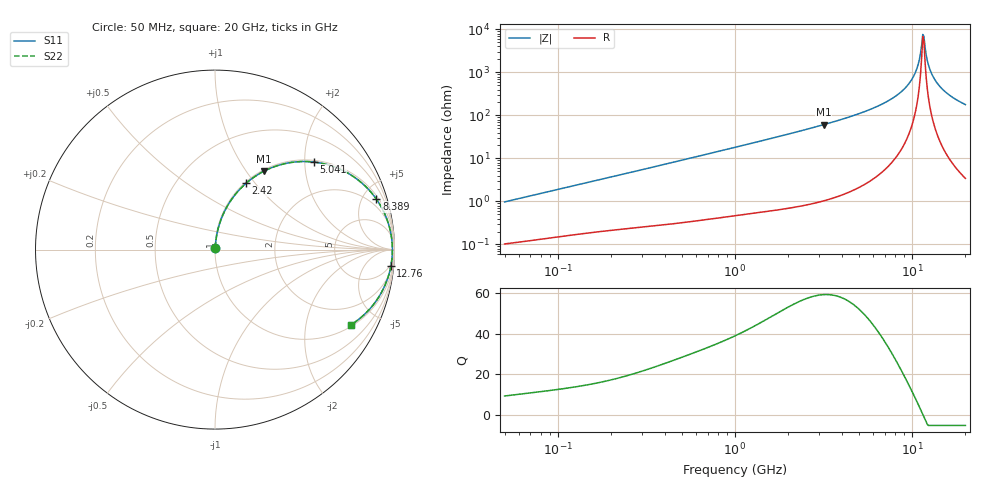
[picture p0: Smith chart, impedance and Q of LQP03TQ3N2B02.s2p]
!Murata Part Number: LQP03TQ3N2B02
!These Parameters are Measured in Series Mode Connection
!  o--[Z]--o
!Port1  Port2
!  o-------o
!Freq. Start=50[MHz] Stop=20[GHz], 401[Steps]
# Hz S RI R 50
!Freq.(Hz) S11(Real) S11(Imag) S21(Real) S21(Imag) S12(Real) S12(Imag) S22(Real) S22(Imag)
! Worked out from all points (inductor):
!   401 points, 50 MHz to 20 GHz, reference 50 ohm
!   read as one part in series: L = 3.07 nH near 51.52 MHz
!   highest Q = 59.1 at 3.169 GHz (marker M1), where L = 3.06 nH
!   self-resonance near 11.49 GHz
!   S11 on the Smith chart (normalised r, x): 50 MHz: 1.00, +0.02; 2.42 GHz: 1.02, +0.90; 5.041 GHz: 1.04, +2.21; 8.389 GHz: 1.26, +6.29; 12.76 GHz: 3, -20; 20 GHz: 1.07, -3.57
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5e7  0.00112 0.0097  0.9989 -0.0097  0.9989 -0.0097  0.00112 0.0097
1.364002e8  0.00242 0.0254  0.9976 -0.0254  0.9976 -0.0254  0.00242 0.0254
3.721004e8  0.00733 0.0672  0.9927 -0.0672  0.9927 -0.0672  0.00733 0.0672
1e9  0.0359 0.1737  0.9641 -0.1737  0.9641 -0.1737  0.0359 0.1737
2.419936e9  0.1734 0.3699  0.8266 -0.3699  0.8266 -0.3699  0.1734 0.3699
2.728004e9  0.2134 0.4012  0.7866 -0.4012  0.7866 -0.4012  0.2134 0.4012
3.168813e9  0.2746 0.4379  0.7254 -0.4379  0.7254 -0.4379  0.2746 0.4379
5.041459e9  0.5498 0.488  0.4502 -0.488  0.4502 -0.488  0.5498 0.488
7.442007e9  0.8286 0.3617  0.1714 -0.3617  0.1714 -0.3617  0.8286 0.3617
8.389408e9  0.899 0.2816  0.101 -0.2816  0.101 -0.2816  0.899 0.2816
9.316812e9  0.9464 0.1977  0.0536 -0.1977  0.0536 -0.1977  0.9464 0.1977
1.019291e10  0.9737 0.1181  0.0263 -0.1181  0.0263 -0.1181  0.9737 0.1181
1.082228e10  0.9842 0.0625  0.0158 -0.0625  0.0158 -0.0625  0.9842 0.0625
1.131968e10  0.9879 0.02  0.0121 -0.02  0.0121 -0.02  0.9879 0.02
1.149051e10  0.9883 0.00574  0.0117 -0.00574  0.0117 -0.00574  0.9883 0.00574
1.183995e10  0.9879 -0.0227  0.0121 0.0227  0.0121 0.0227  0.9879 -0.0227
1.220001e10  0.9859 -0.0511  0.0141 0.0511  0.0141 0.0511  0.9859 -0.0511
1.276073e10  0.9797 -0.0933  0.0203 0.0933  0.0203 0.0933  0.9797 -0.0933
1.375312e10  0.9616 -0.1616  0.0384 0.1616  0.0384 0.1616  0.9616 -0.1616
1.504638e10  0.9278 -0.2381  0.0722 0.2381  0.0722 0.2381  0.9278 -0.2381
1.721783e10  0.8564 -0.3372  0.1436 0.3372  0.1436 0.3372  0.8564 -0.3372
2e10  0.7566 -0.4196  0.2434 0.4196  0.2434 0.4196  0.7566 -0.4196
